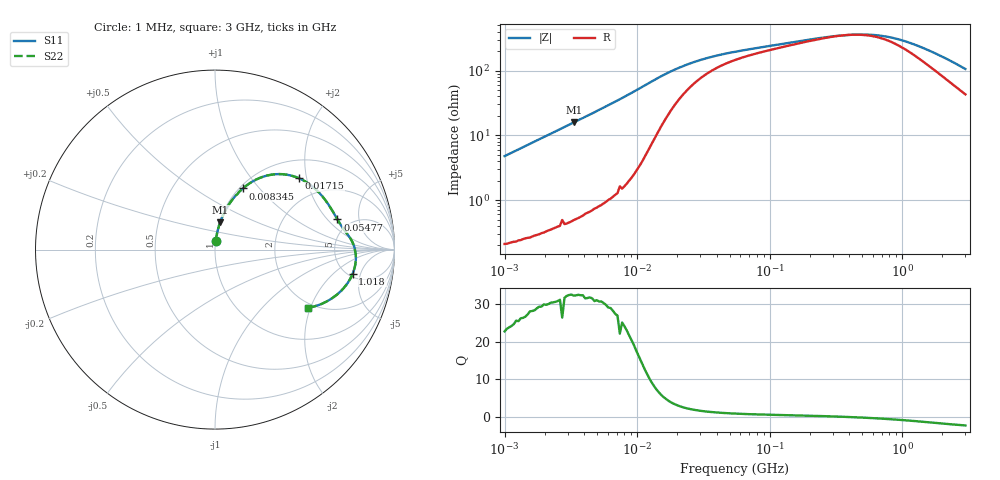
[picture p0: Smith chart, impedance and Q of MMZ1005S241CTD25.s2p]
! S-Parameter Data Generated by TDK Corporation
! Copyright(C) 2025 TDK Corporation.
! All Rights Reserved.
! TDK P/N: MMZ1005S241CTD25 (Chip Bead)
! Property: |Z|=240ohm at 100MHz
! Size(LxWxT): 1x0.5x0.5mm
! Model Type: s2p (Touchstone File Format Version 1.0)
! Frequency: DC=Yes Start=1MHz Stop=3000MHz 202points Log-sweep
! Model Generated on Feb. 6, 2025
! Terms and conditions regarding TDK Simulation Models:
! 1)This simulation model is being provided solely for informational
!  purposes. Please refer to the specifications of the products in
!  terms of detailed characteristics of such products.
! 2)In no event shall TDK Corporation of any of its subsidiaries be
!  liable for any loss or damage arising, directly or indirectly,
!  from any information contained in this simulation model, including,
!  but not limited to loss or damages arising from any inaccuracies,
!  omissions or errors in connection with such information.
! 3)Any and all copyrights on this simulation model are owned by
!  TDK Corporation.  Duplication or redistribution of this simulation
!  model without prior written permission from TDK Corporation
!  is prohibited.
! 4)This simulation model is subject to any modification or change
!  without any prior notice.
! 5)Neither TDK Corporation nor any of its subsidiaries shall make any
!  warranty, express or implied, including but not limited to the
!  correctness, implied warranties of merchantability and fitness for
!  a particular purpose with respect to this simulation models.
! 6)The use of this simulation model shall be deemed to have consented
!  to the terms and conditions hereof.
! Port Assignments:
!  1 ---@@@--- 2
! Applicable Conditions:
!  Temperature = 25 degC
!  DC Bias Current = 0 A
!  Small Signal Operation
# Hz S MA R 50
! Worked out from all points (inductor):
!   201 points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, 1 MHz to 3 GHz, reference 50 ohm
!   read as one part in series: L = 758 nH near 1.041 MHz
!   highest Q = 32.3 at 3.323 MHz (marker M1), where L = 756 nH
!   self-resonance near 388.8 MHz
!   S11 on the Smith chart (normalised r, x): 1 MHz: 1.00, +0.10; 8.345 MHz: 1.04, +0.82; 17.15 MHz: 1.42, +1.81; 54.77 MHz: 3.91, +2.60; 1.018 GHz: 5.45, -3.71; 3 GHz: 1.86, -1.93
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1000000  0.04757 84.8  0.9968 -2.7  0.9968 -2.7  0.04757 84.8
1897447  0.08958 82.9  0.9929 -5.1  0.9929 -5.1  0.08958 82.9
3323290  0.1552 79.3  0.9831 -8.9  0.9831 -8.9  0.1552 79.3
3900413  0.1815 77.8  0.9778 -10.5  0.9778 -10.5  0.1815 77.8
5820586  0.2668 72.6  0.9548 -15.5  0.9548 -15.5  0.2668 72.6
8345207  0.3747 65.5  0.911 -22.0  0.911 -22.0  0.3747 65.5
1.149534e7  0.4938 55.9  0.8307 -29.5  0.8307 -29.5  0.4938 55.9
1.461624e7  0.5757 46.6  0.7346 -34.7  0.7346 -34.7  0.5757 46.6
1.71545e7  0.615 40.2  0.6624 -36.8  0.6624 -36.8  0.615 40.2
2.181181e7  0.6505 31.8  0.5634 -37.5  0.5634 -37.5  0.6505 31.8
2.773354e7  0.6711 25.1  0.4852 -36.0  0.4852 -36.0  0.6711 25.1
5.477226e7  0.7022 13.9  0.36 -27.9  0.36 -27.9  0.7022 13.9
2.136344e8  0.7608 4.1  0.2473 -12.8  0.2473 -12.8  0.7608 4.1
3.453811e8  0.7772 0.9  0.2232 -3.1  0.2232 -3.1  0.7772 0.9
4.75755e8  0.7842 -1.6  0.2173 5.9  0.2173 5.9  0.7842 -1.6
6.296259e8  0.7867 -4.2  0.223 14.9  0.223 14.9  0.7867 -4.2
8.005644e8  0.7852 -6.8  0.2391 22.9  0.2391 22.9  0.7852 -6.8
1.017911e9  0.7785 -9.9  0.2689 29.9  0.2689 29.9  0.7785 -9.9
1.347129e9  0.7615 -14.3  0.3224 35.6  0.3224 35.6  0.7615 -14.3
1.782824e9  0.7296 -19.5  0.3962 38.0  0.3962 38.0  0.7296 -19.5
2.266846e9  0.6868 -24.8  0.4745 37.5  0.4745 37.5  0.6868 -24.8
3e9  0.6125 -32.0  0.58 34.0  0.58 34.0  0.6125 -32.0
